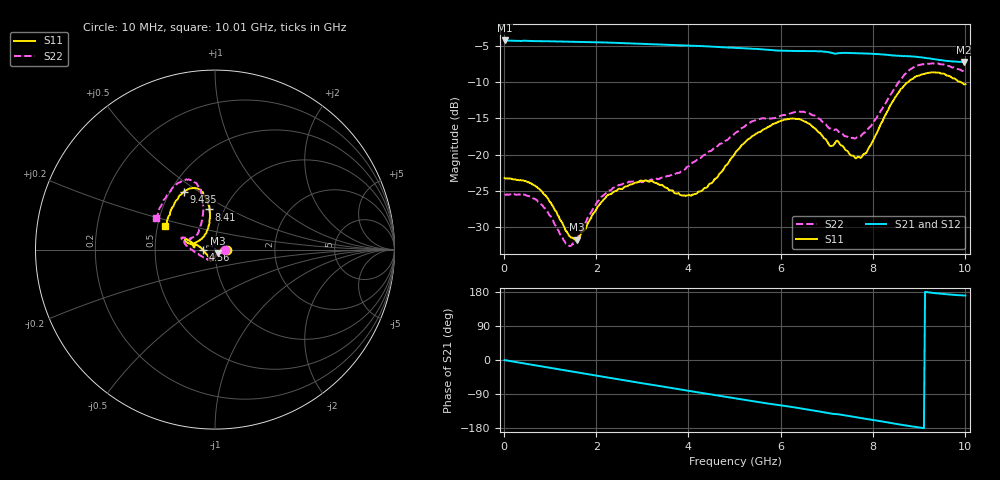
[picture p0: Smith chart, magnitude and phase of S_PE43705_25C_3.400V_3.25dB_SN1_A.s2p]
! Device ID: PE43705
! Serial: 1
! Insertion: A
! Impedance: 50 ohm
! Temp: 25C
! VDD: 3.400V
! Attenuation Step: 3.25dB
#  Hz  S  RI  R  50
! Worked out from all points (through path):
!   401 points, 10 MHz to 10.01 GHz, reference 50 ohm
!   highest |S21| = -4.29 dB at 10 MHz (marker M1); lowest = -7.3 dB at 9.985 GHz (marker M2)
!   group delay of S21, straight-line fit = 54 ps
!   lowest |S11| = -31.7 dB at 1.585 GHz (marker M3), VSWR 1.05, Z = 51.6 - j2.09 ohm
!   |S11| at or under -10 dB: start of sweep to 8.768 GHz; 9.905 GHz to end of sweep
!   |S22| runs from -32.6 to -7.4 dB; largest |S21 - S12| = 0.0047
!   S11 on the Smith chart (normalised r, x): 10 MHz: 1.15, -0.00; 4.56 GHz: 0.87, -0.01; 8.41 GHz: 0.85, +0.40; 9.435 GHz: 0.58, +0.44; 10.01 GHz: 0.55, +0.16
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1e7  0.0692 -0.000304  0.6102 -0.00298  0.6106 -0.00288  0.0535 -9.19e-05
7.35e8  0.0569 0.0151  0.5823 -0.1592  0.5825 -0.1589  0.0452 0.014
1.36e9  0.0286 -0.00759  0.5291 -0.2821  0.5291 -0.2819  0.0221 -0.0105
1.585e9  0.0164 -0.0203  0.5024 -0.3225  0.5026 -0.3225  0.012 -0.0236
1.685e9  0.0118 -0.0269  0.4902 -0.3398  0.4902 -0.3397  0.00647 -0.0298
2.26e9  -0.0101 -0.052  0.4063 -0.4278  0.4064 -0.4274  -0.0175 -0.0535
2.96e9  -0.0244 -0.0617  0.2839 -0.5048  0.2841 -0.5045  -0.0359 -0.0544
3.36e9  -0.0263 -0.0567  0.21 -0.5329  0.2105 -0.5325  -0.0422 -0.0535
3.985e9  -0.0416 -0.0321  0.0882 -0.5565  0.0886 -0.5557  -0.0732 -0.0386
4.56e9  -0.0675 -0.00288  -0.0229 -0.5513  -0.0215 -0.5512  -0.1106 -0.0157
5.01e9  -0.0991 0.0248  -0.1046 -0.5325  -0.1041 -0.5328  -0.1403 0.00662
6.035e9  -0.162 0.0577  -0.2612 -0.4482  -0.2591 -0.4488  -0.1788 0.0547
6.685e9  -0.1523 0.0374  -0.3493 -0.3787  -0.3494 -0.3784  -0.1747 0.0676
7.085e9  -0.113 0.0196  -0.3925 -0.3157  -0.393 -0.3164  -0.1399 0.0576
7.685e9  -0.0691 0.068  -0.4402 -0.2357  -0.4395 -0.2361  -0.0955 0.0931
7.91e9  -0.0464 0.1012  -0.4537 -0.1977  -0.4539 -0.2006  -0.0829 0.1275
8.36e9  -0.0283 0.2103  -0.469 -0.1214  -0.4678 -0.1232  -0.0658 0.2432
8.41e9  -0.0321 0.2236  -0.4691 -0.1128  -0.4684 -0.1136  -0.067 0.2565
8.86e9  -0.077 0.324  -0.4719 -0.0374  -0.4689 -0.0397  -0.1158 0.3765
9.435e9  -0.1739 0.3232  -0.4472 0.0359  -0.4463 0.0364  -0.2142 0.3635
9.985e9  -0.2689 0.1415  -0.4272 0.0736  -0.4279 0.0732  -0.3207 0.1884
1.001e10  -0.2759 0.1314  -0.4284 0.0754  -0.4297 0.0742  -0.3279 0.1766
